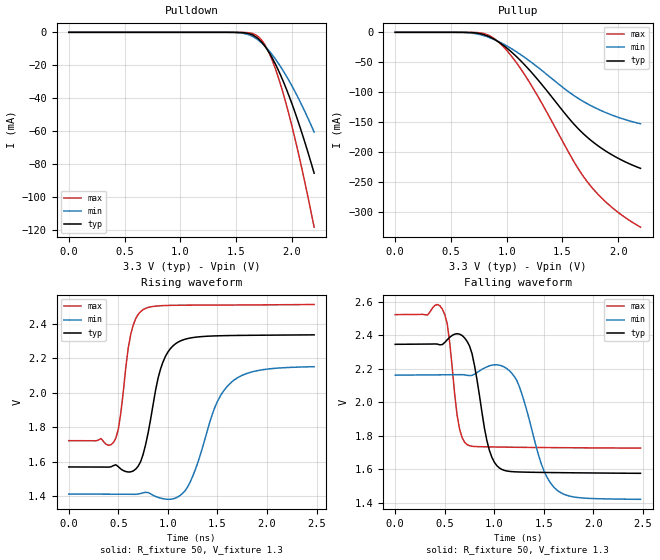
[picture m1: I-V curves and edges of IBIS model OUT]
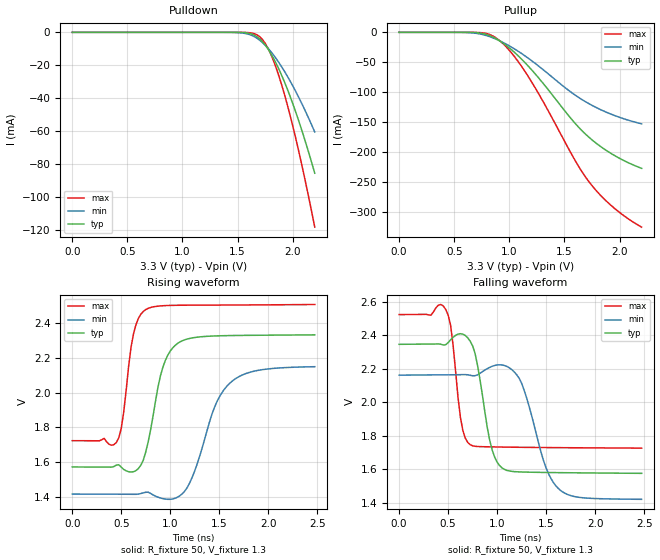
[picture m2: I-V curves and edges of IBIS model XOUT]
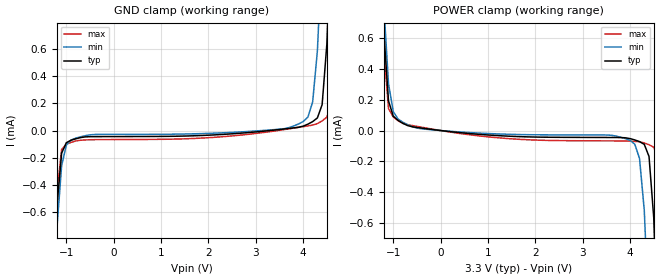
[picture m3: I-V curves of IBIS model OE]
[IBIS Ver]   3.2
[Comment Char]   |_char
[File name]   vg5032edn.ibs
[File Rev]   1.0
[Date]   2015/07/08 5:24:35
[Source]
[Notes]
[Disclaimer]
Seiko Epson Corporation makes no warranty with respect to the information
contained herein.
[Copyright]
Copyright(C) 2014, Seiko Epson Corporation. All rights reserved.
[Component]   vg5032edn
Si_location Pin
Timing_location Pin
[Manufacturer]   Seiko Epson Corporation
[Package]
R_pkg   0.36   NA   NA
L_pkg   4.00n   NA   NA
C_pkg   0.42p   NA   NA
[Pin] signal_name   model_name   R_pin   L_pin   C_pin
1   VC   NC
2   OE   OE   0.10   2.00n   0.77p
3   GND   GND
4   OUT   OUT   0.43   4.00n   0.47p
5   XOUT   XOUT   0.28   4.00n   0.38p
6   VCC   POWER
[Diff Pin] inv_pin vdiff   tdelay_typ
4   5   0   0
| Models and submodels in the file (3): OUT (Output_ECL), XOUT (Output_ECL), OE (Input)
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[Model]   OUT
Model_type Output_ECL
Enable Active-High
Polarity Non-Inverting
Vref=1.3
Vmeas=2
Rref=50
Cref=0
C_comp   0.1p   0.1p   0.1p
[Temperature Range] 25   85   -40
[Voltage Range]   3.3   3.135   3.465
[Pullup Reference]  3.3   3.135   3.465
[Pulldown Reference]3.3   3.135   3.465
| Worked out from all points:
|   falling waveform, R_fixture 50, V_fixture 1.3: 20-80 % time 135ps typ, 221ps min, 87.5ps max; typ from 2.35 V to 1.58 V
|   rising waveform, R_fixture 50, V_fixture 1.3: 20-80 % time 170ps typ, 273ps min, 108ps max; typ from 1.57 V to 2.33 V
[Pullup]
0V        65.87pA    67.75pA    68.98pA
725mV     -1.107mA   -2.446mA   -345.2uA
825mV     -5.887mA   -7.453mA   -3.954mA
900mV     -12.93mA   -13.11mA   -12.17mA
1.025V    -30.05mA   -25.37mA   -35.71mA
1.175V    -57.25mA   -43.82mA   -75.01mA
1.325V    -89.65mA   -65.29mA   -122.1mA
1.6V      -153mA     -105.4mA   -215.5mA
1.725V    -176mA     -119.7mA   -250.7mA
1.825V    -190.7mA   -129.1mA   -272.3mA
1.925V    -202.9mA   -137.1mA   -290mA
2.2V      -227.6mA   -153.1mA   -326mA
[Pulldown]
0V        65.87pA    67.52pA    68.98pA
1.475V    -18.81uA   -96.55uA   -1.663uA
1.625V    -1.007mA   -1.782mA   -394.6uA
1.7V      -3.967mA   -4.778mA   -2.647mA
1.75V     -7.671mA   -7.813mA   -6.661mA
1.8V      -12.73mA   -11.59mA   -13.11mA
1.85V     -18.96mA   -16.01mA   -21.68mA
1.925V    -30.17mA   -23.7mA    -37.74mA
1.975V    -38.72mA   -29.46mA   -50.18mA
2.05V     -52.97mA   -38.95mA   -70.98mA
2.125V    -68.7mA    -49.39mA   -93.91mA
2.2V      -85.73mA   -60.68mA   -118.6mA
[Falling Waveform]
R_fixture=50
V_fixture=1.3
V_fixture_min=1.135
V_fixture_max=1.465
0s        2.346V     2.163V     2.524V
475ps     2.345V     2.164V     2.557V
525ps     2.374V     2.165V     2.469V
650ps     2.407V     2.166V     1.839V
725ps     2.364V     2.161V     1.748V
925ps     1.771V     2.212V     1.735V
1.05ns    1.609V     2.222V     1.733V
1.225ns   1.585V     2.133V     1.732V
1.625ns   1.581V     1.48V      1.73V
2.475ns   1.577V     1.422V     1.727V
[Rising Waveform]
R_fixture=50
V_fixture=1.3
V_fixture_min=1.135
V_fixture_max=1.465
0s        1.571V     1.414V     1.723V
450ps     1.579V     1.413V     1.712V
500ps     1.572V     1.413V     1.79V
625ps     1.542V     1.413V     2.337V
750ps     1.644V     1.421V     2.48V
925ps     2.136V     1.39V      2.503V
1.075ns   2.282V     1.391V     2.505V
1.225ns   2.316V     1.484V     2.506V
1.625ns   2.33V      2.052V     2.507V
2.475ns   2.334V     2.15V      2.51V
[Ramp]
R_load=50
dV/dt_r   4.668e-1/1.840e-10   4.818e-1/2.887e-10   4.812e-1/1.155e-10
dV/dt_f   4.668e-1/1.430e-10   4.818e-1/2.327e-10   4.812e-1/8.994e-11
|[End   OUT
[Model]   XOUT
Model_type Output_ECL
Enable Active-High
Polarity Inverting
Vref=1.3
Vmeas=2
Rref=50
Cref=0
C_comp   0.1p   0.1p   0.1p
[Model Spec]
[Temperature Range] 25   85   -40
[Voltage Range]   3.3   3.135   3.465
[Pullup Reference]  3.3   3.135   3.465
[Pulldown Reference]3.3   3.135   3.465
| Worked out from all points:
|   falling waveform, R_fixture 50, V_fixture 1.3: 20-80 % time 135ps typ, 221ps min, 87.5ps max; typ from 2.35 V to 1.58 V
|   rising waveform, R_fixture 50, V_fixture 1.3: 20-80 % time 169ps typ, 274ps min, 108ps max; typ from 1.57 V to 2.33 V
[Pullup]
0V        65.87pA    67.75pA    68.98pA
725mV     -1.107mA   -2.446mA   -345.2uA
825mV     -5.887mA   -7.453mA   -3.954mA
900mV     -12.93mA   -13.11mA   -12.17mA
1.025V    -30.05mA   -25.37mA   -35.71mA
1.175V    -57.25mA   -43.82mA   -75.01mA
1.325V    -89.65mA   -65.29mA   -122.1mA
1.6V      -153mA     -105.4mA   -215.5mA
1.725V    -176mA     -119.7mA   -250.7mA
1.825V    -190.7mA   -129.1mA   -272.3mA
1.925V    -202.9mA   -137.1mA   -290mA
2.2V      -227.6mA   -153.1mA   -326mA
[Pulldown]
0V        65.87pA    67.52pA    68.98pA
1.475V    -18.81uA   -96.55uA   -1.663uA
1.625V    -1.007mA   -1.782mA   -394.6uA
1.7V      -3.967mA   -4.778mA   -2.647mA
1.75V     -7.671mA   -7.813mA   -6.661mA
1.8V      -12.73mA   -11.59mA   -13.11mA
1.85V     -18.96mA   -16.01mA   -21.68mA
1.925V    -30.17mA   -23.7mA    -37.74mA
1.975V    -38.72mA   -29.46mA   -50.18mA
2.05V     -52.97mA   -38.95mA   -70.98mA
2.125V    -68.7mA    -49.39mA   -93.91mA
2.2V      -85.73mA   -60.68mA   -118.6mA
[Falling Waveform]
R_fixture=50
V_fixture=1.3
V_fixture_min=1.135
V_fixture_max=1.465
0s        2.346V     2.162V     2.523V
475ps     2.344V     2.164V     2.555V
525ps     2.373V     2.165V     2.461V
625ps     2.41V      2.165V     1.912V
725ps     2.365V     2.162V     1.748V
925ps     1.773V     2.209V     1.735V
1.05ns    1.609V     2.223V     1.734V
1.25ns    1.585V     2.114V     1.732V
1.625ns   1.581V     1.486V     1.73V
2.475ns   1.577V     1.422V     1.727V
[Rising Waveform]
R_fixture=50
V_fixture=1.3
V_fixture_min=1.135
V_fixture_max=1.465
0s        1.571V     1.414V     1.723V
450ps     1.581V     1.413V     1.713V
500ps     1.569V     1.413V     1.794V
625ps     1.543V     1.413V     2.34V
750ps     1.657V     1.425V     2.481V
925ps     2.148V     1.388V     2.503V
1.075ns   2.285V     1.396V     2.505V
1.2ns     2.314V     1.481V     2.506V
1.6ns     2.33V      2.051V     2.507V
2.475ns   2.334V     2.15V      2.51V
[Ramp]
R_load=50
dV/dt_r   4.668E-1/1.808E-10   4.818E-1/2.887E-10   4.812E-1/1.159E-10
dV/dt_f   4.668E-1/1.422E-10   4.818E-1/2.319E-10   4.812E-1/9.081E-11
|[End   XOUT
[Model]   OE
Model_type Input
Vinh=2.31
Vinl=0.99
C_comp   2p   2p   2p
[Model Spec]
[Temperature Range] 25   85   -40
[Voltage Range]   3.3   3.135   3.465
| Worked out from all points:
|   GND clamp passes 1 mA (typ) near -1.25 V on its own axis
|   POWER clamp passes 1 mA (typ) near -1.24 V on its own axis
[GND Clamp]
-3.3V     -24.59mA   -20.9mA    -29.61mA
-1.3V     -1.492mA   -1.552mA   -1.557mA
-1.2V     -564.6uA   -724.3uA   -469.2uA
-1.1V     -167.5uA   -259uA     -139.5uA
-900mV    -71.67uA   -70.02uA   -87.5uA
3.9V      24.29uA    48.34uA    23.21uA
4.2V      65.85uA    211.8uA    40.14uA
4.3V      93.27uA    590uA      51.34uA
4.4V      191.4uA    1.349mA    71.39uA
4.6V      1.622mA    3.351mA    204.2uA
4.7V      2.825mA    4.361mA    851.7uA
6.6V      25.83mA    23.65mA    28.68mA
[POWER Clamp]
-3.3V     25.83mA    21.96mA    31.12mA
-1.3V     1.622mA    1.685mA    1.684mA
-1.2V     640.5uA    815.4uA    526.2uA
-1.1V     191.4uA    302.3uA    141.8uA
-700mV    32.36uA    38.59uA    37.98uA
4V        -52.14uA   -64.11uA   -68.59uA
4.2V      -71.67uA   -181.2uA   -72.81uA
4.4V      -167.5uA   -1.229mA   -91.72uA
4.5V      -564.6uA   -2.178mA   -107.9uA
4.6V      -1.492mA   -3.141mA   -189.7uA
4.7V      -2.641mA   -4.106mA   -767.5uA
6.6V      -24.59mA   -22.51mA   -27.29mA
